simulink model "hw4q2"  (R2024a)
settings: Solver=VariableStepAuto  StartTime=0.0  StopTime=20  MaxStep=0.0001  RelTol=1e-3

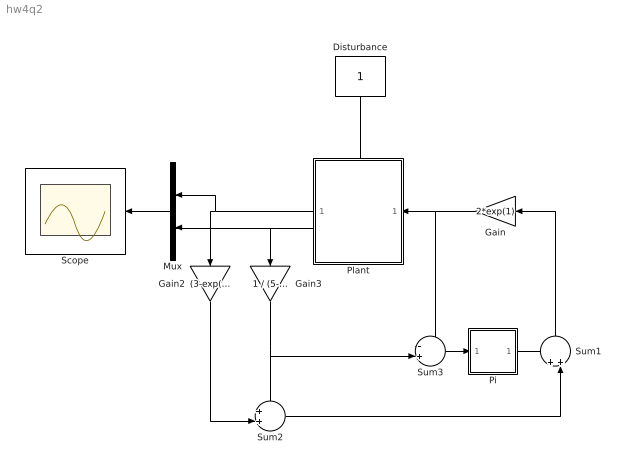
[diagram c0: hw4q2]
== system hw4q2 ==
  Disturbance : Constant
  Gain : Gain  Gain=2*exp(1)
  Gain2 : Gain  Gain=(3-exp(-1)) / (5-2*exp(-1))
  Gain3 : Gain  Gain=1 / (5-2*exp(-1))
  Mux : Mux  Inputs=2
  Pi : Subsystem
  Plant : Subsystem
  Scope : Scope
  Sum1 : Sum  Inputs=++|
  Sum2 : Sum  Inputs=++|
  Sum3 : Sum  Inputs=-+|
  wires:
  Mux/1 -> Scope/1
  Disturbance/1 -> Plant/2(In1)
  Plant/1(Out1) -> Mux/1, Gain2/1
  Plant/2(Out2) -> Gain3/1, Mux/2
  Gain/1 -> Sum3/1, Plant/1(In2)
  Sum1/1 -> Gain/1
  Gain3/1 -> Sum2/1, Sum3/2
  Gain2/1 -> Sum2/2
  Sum2/1 -> Sum1/2
  Sum3/1 -> Pi/1(In1)
  Pi/1(Out1) -> Sum1/1

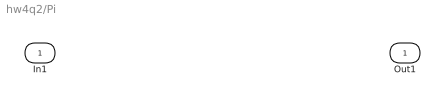
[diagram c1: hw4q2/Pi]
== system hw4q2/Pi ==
  In1 : Inport
  Out1 : Outport

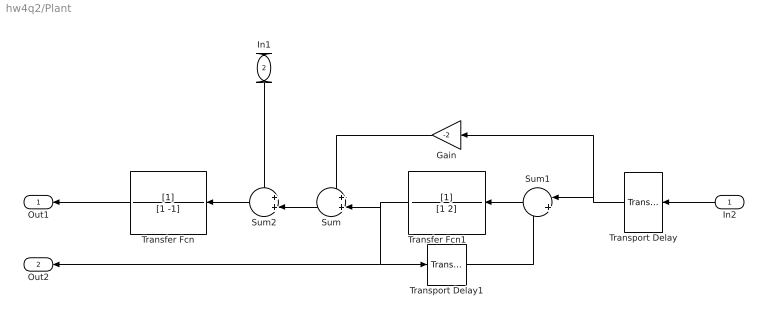
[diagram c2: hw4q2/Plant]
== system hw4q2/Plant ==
  In2 : Inport
  In1 : Inport  Port=2
  Gain : Gain  Gain=-2
  Sum : Sum  Inputs=++|
  Sum1 : Sum  Inputs=|++
  Sum2 : Sum  Inputs=++|
  Transfer Fcn : TransferFcn  Denominator=[1 -1]
  Transfer Fcn1 : TransferFcn  Denominator=[1 2]
  Transport Delay : TransportDelay
  Transport Delay1 : TransportDelay
  Out1 : Outport
  Out2 : Outport  Port=2
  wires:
  In2/1 -> Transport Delay/1
  Transfer Fcn/1 -> Out1/1
  In1/1 -> Sum2/1
  Transport Delay1/1 -> Sum1/2
  Sum1/1 -> Transfer Fcn1/1
  Sum2/1 -> Transfer Fcn/1
  Gain/1 -> Sum/1
  Transfer Fcn1/1 -> Out2/1, Transport Delay1/1, Sum/2
  Transport Delay/1 -> Gain/1, Sum1/1
  Sum/1 -> Sum2/2
